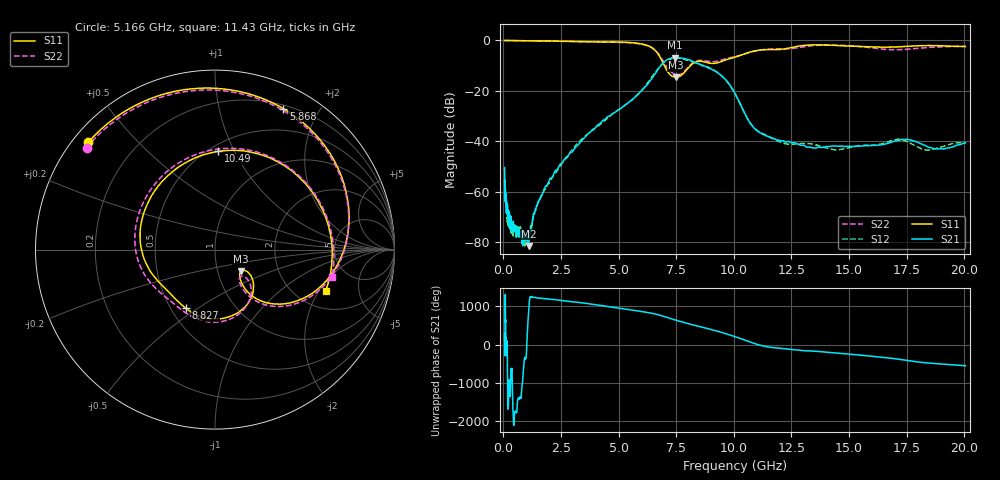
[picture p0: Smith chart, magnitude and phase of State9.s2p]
# Hz S DB R 50
!freq MagS11 AngS11 MagS21 AngS21 MagS12 AngS12 MagS22 AngS22
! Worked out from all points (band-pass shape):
!   1601 points, 50 MHz to 20.05 GHz, reference 50 ohm
!   highest |S21| = -6.81 dB at 7.458 GHz (marker M1); lowest = -81.5 dB at 1.087 GHz (marker M2)
!   |S21| within 3 dB of the highest: 6.844 GHz to 8.586 GHz (1.742 GHz wide, 22.6 % of centre)
!   lowest |S11| = -14.6 dB at 7.486 GHz (marker M3), VSWR 1.46, Z = 64.5 - j16 ohm
!   |S11| at or under -10 dB: 6.983 GHz to 8.111 GHz (1.128 GHz wide, 15 % of centre)
!   |S22| runs from -13.7 to 0.0 dB; largest |S21 - S12| = 0.024
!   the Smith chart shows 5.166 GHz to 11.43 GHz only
!   S11 on the Smith chart (normalised r, x): 5.166 GHz: 0.04, +0.37; 5.868 GHz: 0.24, +1.57; 8.827 GHz: 0.60, -0.45; 10.49 GHz: 0.55, +0.87; 11.43 GHz: 2.84, -2.30
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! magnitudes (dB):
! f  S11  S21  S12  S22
! 50 MHz  0.0  -50.4  -55.0  0.0
! 77.21 MHz  0.0  -60.9  -57.6  0.0
! 81.68 MHz  0.0  -63.3  -63.0  0.0
! 135.9 MHz  0.0  -64.4  -64.9  0.0
! 164 MHz  0.0  -67.9  -71.9  0.0
! 369.6 MHz  0.0  -75.0  -74.5  0.0
! 1.005 GHz  -0.1  -78.7  -77.6  -0.1
! 1.087 GHz  -0.1  -81.5  -77.3  -0.1
! 1.462 GHz  -0.2  -65.3  -65.4  -0.2
! 2.722 GHz  -0.3  -46.7  -46.4  -0.4
! 5.166 GHz  -0.7  -26.4  -26.3  -0.8
! 5.868 GHz  -1.2  -21.1  -21.1  -1.3
! 6.541 GHz  -3.6  -13.7  -13.2  -3.5
! 7.402 GHz  -14.5  -6.8  -7.1  -13.2
! 7.458 GHz  -14.5  -6.8  -7.1  -13.5
! 7.486 GHz  -14.6  -6.8  -7.1  -13.6
! 8.827 GHz  -8.8  -10.6  -10.4  -8.2
! 9.694 GHz  -7.6  -16.0  -16.3  -7.2
! 10.49 GHz  -5.2  -29.2  -29.2  -5.3
! 11.43 GHz  -3.6  -37.9  -37.7  -3.5
! 14.37 GHz  -1.9  -41.9  -43.4  -1.9
! 20.05 GHz  -2.4  -40.7  -40.5  -2.4
